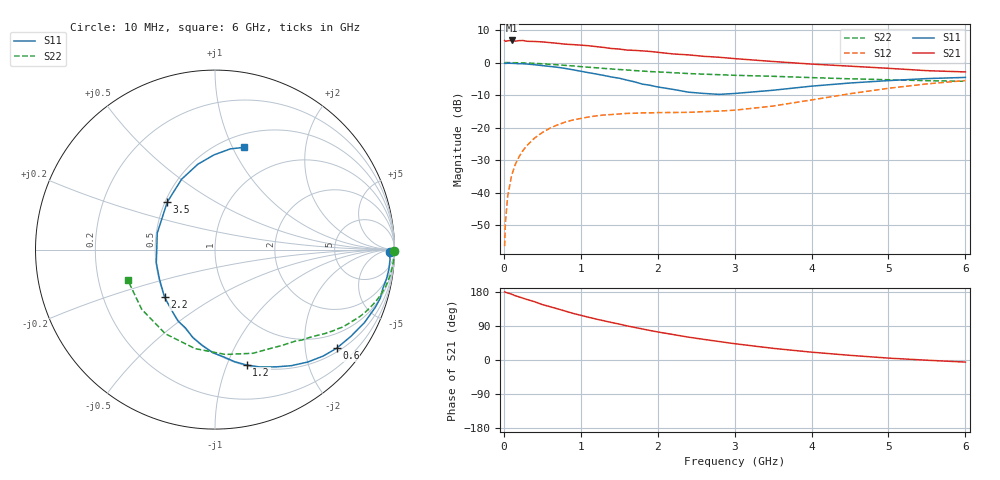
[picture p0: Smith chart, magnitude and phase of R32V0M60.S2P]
! SIEMENS Small Signal Semiconductors
! BFR181
! Si NPN RF Bipolar Junction Transistor in SOT23
! VCE = 2 V  IC = 0.6 mA
! Common Emitter S-Parameters:  May  1996
# GHz  S  MA  R  50
!  f  S11  S21  S12  S22
! GHz  MAG  ANG  MAG  ANG  MAG  ANG  MAG  ANG
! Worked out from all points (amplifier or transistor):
!   36 points, 10 MHz to 6 GHz, reference 50 ohm
!   highest |S21| = 6.8 dB at 100 MHz (marker M1)
!   |S21| within 3 dB of that: start of sweep to 1.646 GHz
!   unconditionally stable (mu >= 1): 2.254 GHz to 3.908 GHz
!   at 250 MHz: K = 0.13, MSG = 16.9 dB, |S12| = -27.0 dB
!   at 1.4 GHz: K = 0.66, MSG = 10.2 dB, |S12| = -16.0 dB
!   at 6 GHz: K = 0.91, MSG = 1.3 dB, |S12| = -5.5 dB
!   S11 on the Smith chart (normalised r, x): 10 MHz: 63, -37; 600 MHz: 0.59, -2.70; 1.2 GHz: 0.51, -1.18; 2.2 GHz: 0.50, -0.31; 3.5 GHz: 0.51, +0.32; 6 GHz: 0.63, +1.10
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0.01  0.9766 -0.8  2.184 179.7  0.0015 91.4  0.9994 -0.4
0.02  0.971 -1.4  2.123 178.6  0.0034 86.4  0.9989 -0.7
0.05  0.977 -3.2  2.163 176.9  0.0088 87.7  0.9988 -1.6
0.1  0.975 -6.5  2.189 173.8  0.0182 85.7  0.9971 -3.1
0.15  0.9695 -9.6  2.139 169.5  0.0274 82.5  0.9946 -4.7
0.2  0.9597 -13.1  2.178 166.4  0.036 80.9  0.9909 -6.2
0.25  0.9596 -16.5  2.184 163.1  0.0446 78.4  0.9881 -7.8
0.3  0.9492 -19.8  2.128 159.7  0.0529 76.5  0.9832 -9.3
0.5  0.8984 -32.5  2.08 146.3  0.084 68.3  0.9582 -15.1
0.6  0.8723 -39.1  2.029 140.7  0.0981 64.1  0.9415 -17.8
0.9  0.7739 -56.7  1.889 123.0  0.1309 53.6  0.8875 -25.0
1.1  0.6999 -69.1  1.816 112.9  0.1455 48.1  0.8485 -29.2
1.2  0.6672 -74.6  1.761 108.0  0.1513 45.4  0.8316 -31.3
1.7  0.5052 -104.2  1.541 86.0  0.1663 37.6  0.7534 -39.0
1.9  0.4476 -117.5  1.484 77.9  0.1682 36.4  0.7274 -41.8
2.2  0.3869 -136.6  1.358 67.2  0.1707 35.6  0.699 -46.1
2.4  0.3505 -152.0  1.314 60.3  0.1715 37.1  0.6777 -48.9
2.8  0.3243 177.6  1.207 48.7  0.1796 40.4  0.6509 -55.2
3.5  0.3754 135.1  1.039 30.8  0.2146 47.6  0.6152 -69.9
4.5  0.4851 101.4  0.881 12.3  0.3321 48.2  0.5627 -101.3
5.5  0.5674 81.4  0.751 -0.6  0.4702 35.6  0.5267 -140.9
6  0.5912 74.4  0.718 -5.5  0.5291 27.1  0.5151 -161.1
